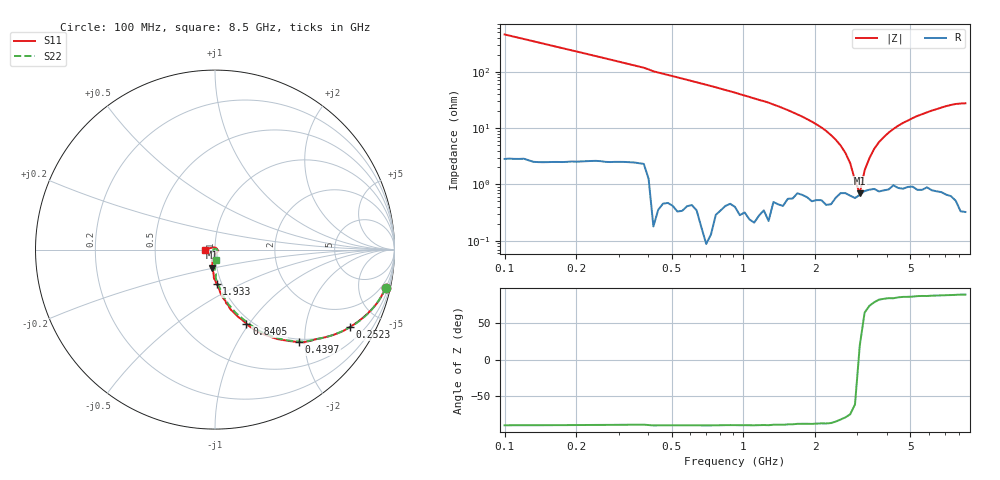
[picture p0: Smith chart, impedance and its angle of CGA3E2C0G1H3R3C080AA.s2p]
! S-parameter Generated by TDK Corporation
! Copyright(C) 2015 TDK Corporation.
! All Rights Reserved.
! TDK P/N: CGA3E2C0G1H3R3C080AA (Multilayer Ceramic Chip Capacitors)
! Property: C=3.3pF
! Size(LxWxT): 1.6x0.8x0.8mm, 0.063x0.031x0.031inches
! Model Type: s2p (Touchstone File Format Version 1.0)
! Frequency: DC=Yes Start=100MHz Stop=8500MHz 98points Log-sweep
! Note:
! Model Generated on Jun. 23, 2015
! Hash(MD5):
! Port Assignments:
!  1 ---| |--- 2
! Applicable Conditions:
!  Temperature = 25 degC
!  DC Bias Voltage = 0 V
!  Small Signal Operation
! Terms and conditions regarding TDK Simulation Models
! (1)This simulation model is being provided solely for informational purposes. Please refer to the specifications of the products in terms of detailed characteristics of such products.
! (2)In no event shall TDK Corporation of any of its subsidiaries be liable for any loss or damage arising, directly or indirectly,
!  From any information contained in this simulation model, including, but not limited to loss or damages arising from any inaccuracies, omissions or errors in connection with such information.
! (3)Any and all copyrights on this simulation model are owned by TDK Corporation.
!  Duplication or redistribution of this simulation model without prior written permission from TDK Corporation is prohibited.
! (4)This simulation model is subject to any modification or change without any prior notice.
! (5)Neither TDK Corporation nor any of its subsidiaries shall make any warranty, express or implied,
!  Including but not limited to the correctness, implied warranties of merchantability and fitness for a particular purpose with respect to this simulation models.
! (6)The use of this simulation model shall be deemed to have consented to the terms and conditions hereof.
# MHz S MA R 50
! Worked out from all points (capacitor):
!   97 points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, 100 MHz to 8.5 GHz, reference 50 ohm
!   read as one part in series: C = 3.48 pF near 100 MHz
!   lowest |Z| = 696 mohm at 3.071 GHz (marker M1)
!   series resonance near 3.045 GHz, so ESL is about 790 pH
!   S11 on the Smith chart (normalised r, x): 100 MHz: 1.02, -8.80; 252.3 MHz: 1.01, -3.47; 439.7 MHz: 0.94, -1.88; 840.5 MHz: 0.94, -0.97; 1.933 GHz: 0.94, -0.37; 8.5 GHz: 0.89, -0.01
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100  0.9746 -12.8  0.2132 76.9  0.2128 77.1  0.9755 -12.7
166.3716  0.9348 -20.8  0.3405 68.9  0.3399 69.1  0.9376 -20.4
252.3262  0.8655 -30.0  0.4788 59.5  0.478 59.7  0.8707 -29.5
439.683  0.6964 -47.7  0.7108 42.6  0.7098 42.8  0.7004 -46.9
636.6849  0.5548 -59.2  0.8262 31.2  0.8249 31.5  0.5554 -58.3
840.4526  0.4489 -67.0  0.8905 23.2  0.8891 23.4  0.4468 -65.9
1533.871  0.2533 -81.8  0.9597 8.4  0.9581 8.7  0.251 -80.5
1933.211  0.1912 -87.5  0.974 3.3  0.9722 3.6  0.1959 -84.9
2931.989  0.1088 -98.9  0.9842 -5.4  0.9823 -5.0  0.1128 -90.9
3070.863  0.1019 -99.8  0.985 -6.3  0.983 -6.0  0.1023 -89.9
3870.357  0.05933 -104.2  0.9866 -11.5  0.9843 -11.1  0.05744 -91.3
4446.777  0.03113 -97.6  0.9858 -14.8  0.9851 -14.5  0.03533 -96.8
5351.035  0.01768 -49.6  0.9873 -20.0  0.9845 -19.4  0.01149 -144.2
5869.945  0.01996 -29.3  0.9873 -22.7  0.9842 -22.4  0.009749 -174.6
6147.976  0.01735 -11.0  0.9855 -24.3  0.9855 -23.8  0.008467 169.1
6439.175  0.01345 -7.6  0.9873 -25.8  0.9842 -25.4  0.005347 154.5
6744.168  0.01171 16.2  0.9863 -27.4  0.9841 -26.9  0.004365 94.7
7063.606  0.01174 61.9  0.9866 -29.0  0.9839 -28.6  0.008401 36.3
7398.175  0.01235 106.5  0.9862 -30.7  0.9839 -30.3  0.01225 -6.0
7748.59  0.01776 138.1  0.9858 -32.7  0.9833 -31.9  0.01905 -33.3
8115.603  0.03419 169.6  0.9854 -34.4  0.9856 -33.8  0.03313 -68.5
8500  0.05701 -175.4  0.9836 -36.5  0.9823 -35.7  0.05564 -82.8
